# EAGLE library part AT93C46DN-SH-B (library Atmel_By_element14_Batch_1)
Three-wire Serial EEPROM
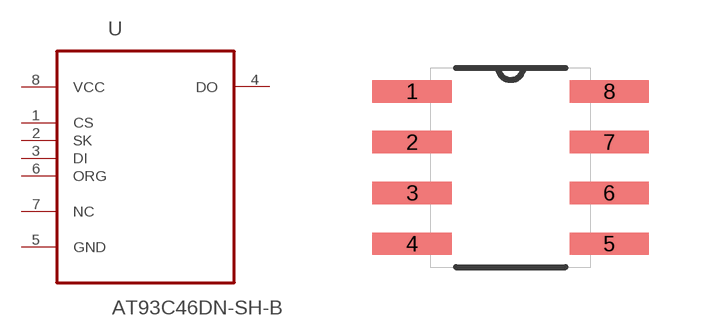
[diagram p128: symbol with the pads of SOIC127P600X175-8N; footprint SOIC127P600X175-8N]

Designator prefix U

## AT93C46DN-SH-B (MPN: AT93C46DN-SH-B; OC_FARNELL: 1455086; OC_NEWARK: 58M3879; PACKAGE: SOIC-8; SUPPLIER: Atmel)  [SOIC127P600X175-8N]
1  CS  in
2  SK  in
3  DI  in
4  DO  out
5  GND  pas
6  ORG  in
7  NC  nc
8  VCC  pwr

## Footprint SOIC127P600X175-8N (pad centres in mm)
smd 1.981 x 0.559: 1 -2.464,1.905; 2 -2.464,0.635; 3 -2.464,-0.635; 4 -2.464,-1.905; 5 2.464,-1.905; 6 2.464,-0.635; 7 2.464,0.635; 8 2.464,1.905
